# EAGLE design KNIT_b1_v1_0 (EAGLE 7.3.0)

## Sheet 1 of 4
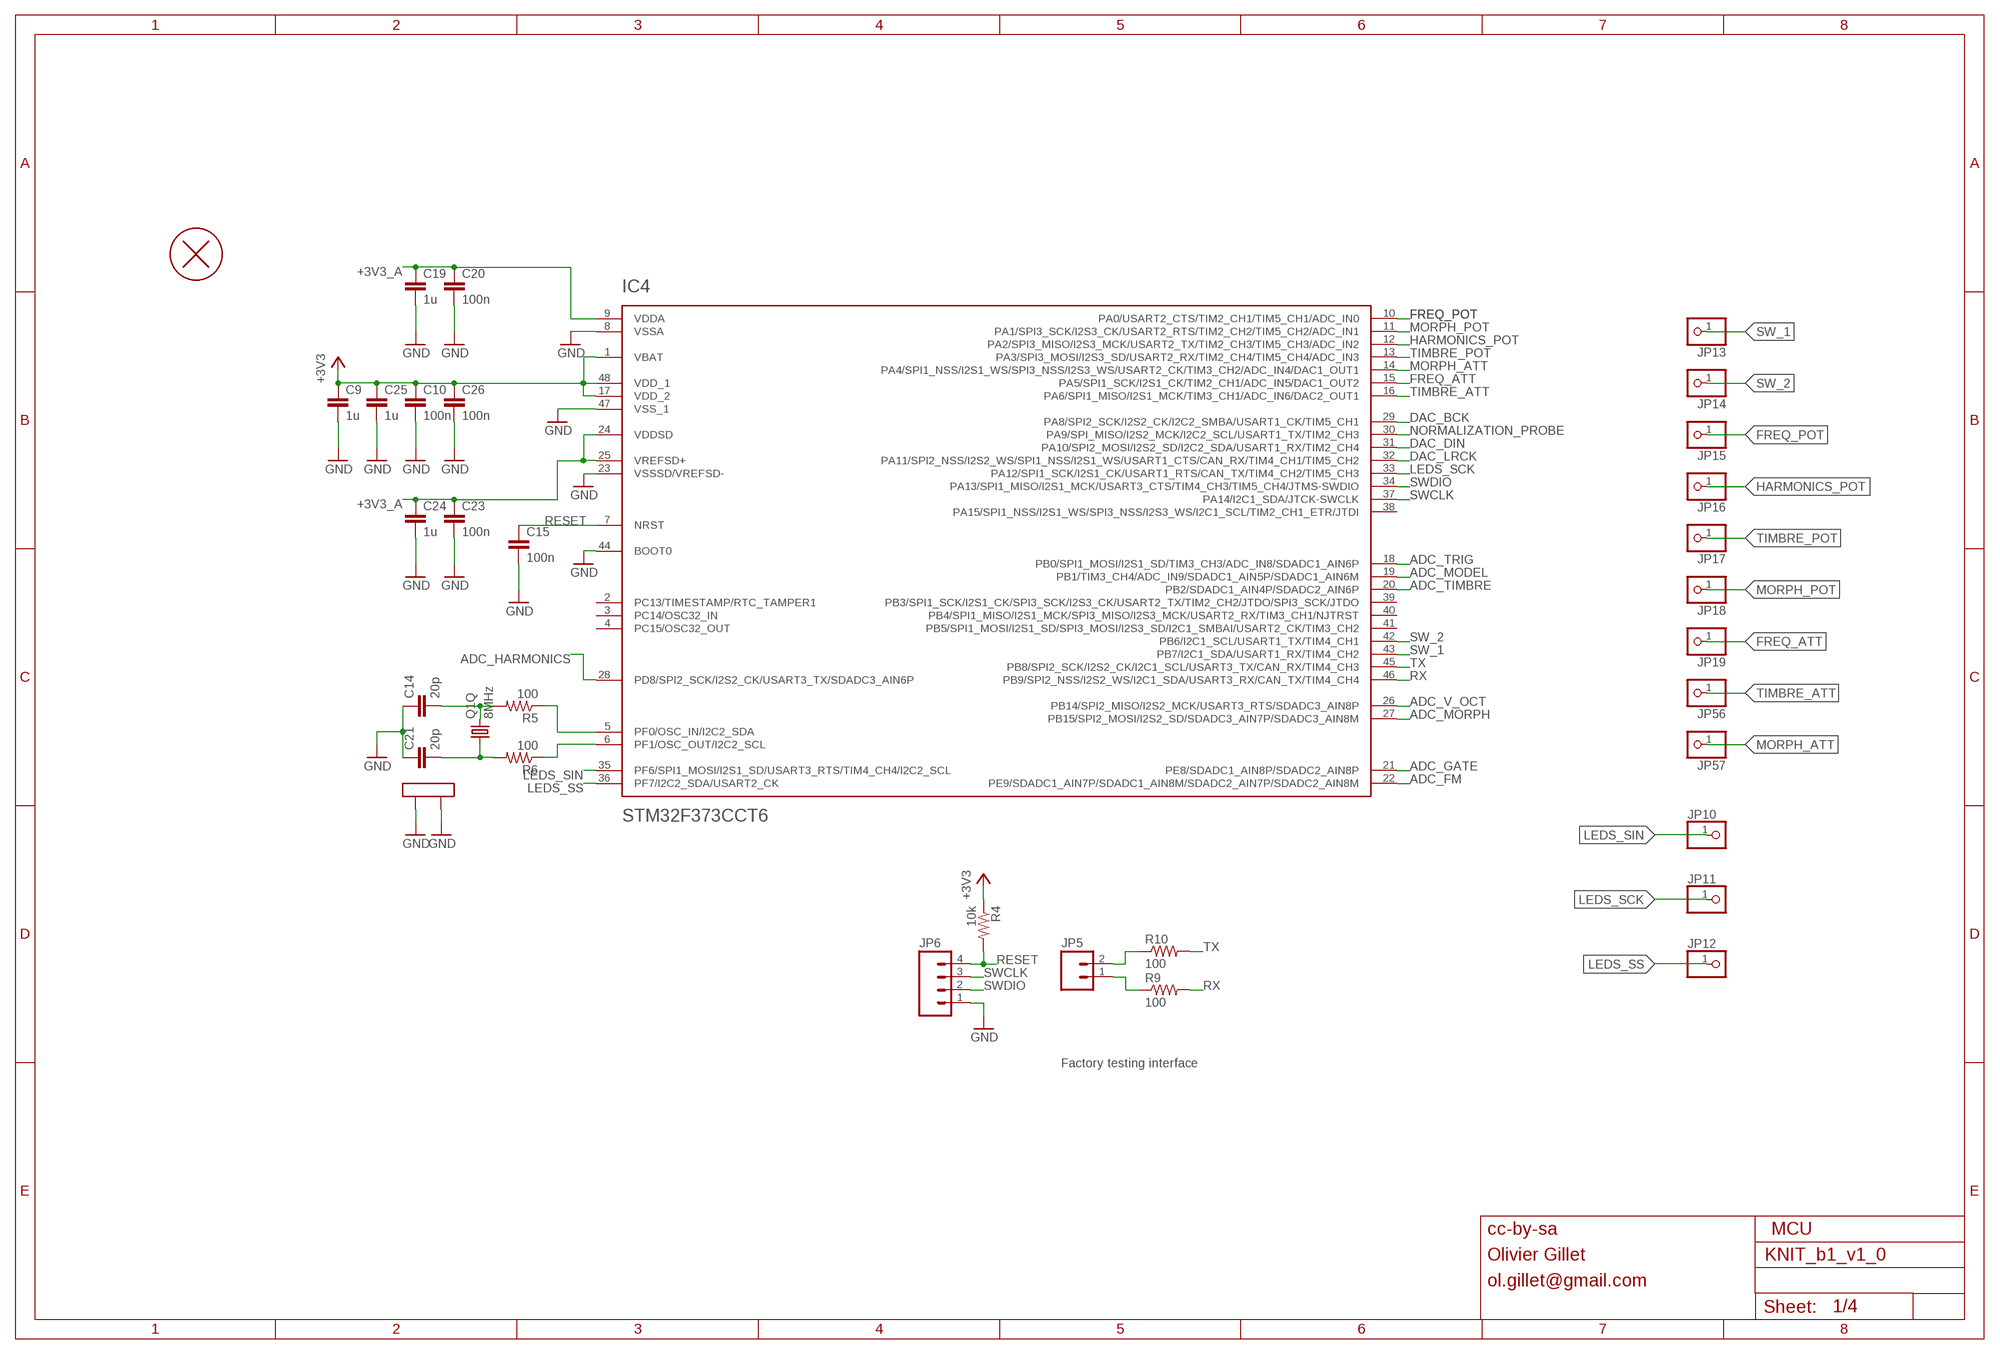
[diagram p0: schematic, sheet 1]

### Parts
C9  1u  CAPACITOR  [RESISTOR_0603]
C10  100n  CAPACITOR  [RESISTOR_0603]
C14  20p  CAPACITOR  [RESISTOR_0603]
C15  100n  CAPACITOR  [RESISTOR_0603]
C19  1u  CAPACITOR  [RESISTOR_0603]
C20  100n  CAPACITOR  [RESISTOR_0603]
C21  20p  CAPACITOR  [RESISTOR_0603]
C23  100n  CAPACITOR  [RESISTOR_0603]
C24  1u  CAPACITOR  [RESISTOR_0603]
C25  1u  CAPACITOR  [RESISTOR_0603]
C26  100n  CAPACITOR  [RESISTOR_0603]
H1  PCB_SCREW  [PCB_SCREW]
IC4  STM32F373CCT6  STM32F373C  [LQFP48]
JP5  M02PTH  [1X02]
JP6  M04PTH  [1X04]
JP10  PINHD-1X1  [1X01]
JP11  PINHD-1X1  [1X01]
JP12  PINHD-1X1  [1X01]
JP13  PINHD-1X1  [1X01]
JP14  PINHD-1X1  [1X01]
JP15  PINHD-1X1  [1X01]
JP16  PINHD-1X1  [1X01]
JP17  PINHD-1X1  [1X01]
JP18  PINHD-1X1  [1X01]
JP19  PINHD-1X1  [1X01]
JP56  PINHD-1X1  [1X01]
JP57  PINHD-1X1  [1X01]
Q1  8MHz  CRYSTAL  [CTS406]
R4  10k  RESISTOR  [RESISTOR_0603]
R5  100  RESISTOR  [RESISTOR_0603]
R6  100  RESISTOR  [RESISTOR_0603]
R9  100  RESISTOR  [RESISTOR_0603]
R10  100  RESISTOR  [RESISTOR_0603]

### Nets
+3V3: C9.1 C10.1 C25.1 C26.1 IC4.1(VBAT) IC4.17(VDD_2) IC4.48(VDD_1) R4.1 ; also sheet 3,4
+3V3_A: C19.1 C20.1 C23.1 C24.1 IC4.9(VDDA) IC4.24(VDDSD) IC4.25(VREFSD+) ; also sheet 2,3,4
ADC_FM: IC4.22(PE9/SDADC1_AIN7P/SDADC1_AIN8M/SDADC2_AIN7P/SDADC2_AIN8M) ; also sheet 2
ADC_GATE: IC4.21(PE8/SDADC1_AIN8P/SDADC2_AIN8P) ; also sheet 2
ADC_HARMONICS: IC4.28(PD8/SPI2_SCK/I2S2_CK/USART3_TX/SDADC3_AIN6P) ; also sheet 2
ADC_MODEL: IC4.19(PB1/TIM3_CH4/ADC_IN9/SDADC1_AIN5P/SDADC1_AIN6M) ; also sheet 2
ADC_MORPH: IC4.27(PB15/SPI2_MOSI/I2S2_SD/SDADC3_AIN7P/SDADC3_AIN8M) ; also sheet 2
ADC_TIMBRE: IC4.20(PB2/SDADC1_AIN4P/SDADC2_AIN6P) ; also sheet 2
ADC_TRIG: IC4.18(PB0/SPI1_MOSI/I2S1_SD/TIM3_CH3/ADC_IN8/SDADC1_AIN6P) ; also sheet 2
ADC_V_OCT: IC4.26(PB14/SPI2_MISO/I2S2_MCK/USART3_RTS/SDADC3_AIN8P) ; also sheet 2
DAC_BCK: IC4.29(PA8/SPI2_SCK/I2S2_CK/I2C2_SMBA/USART1_CK/TIM5_CH1) ; also sheet 3
DAC_DIN: IC4.31(PA10/SPI2_MOSI/I2S2_SD/I2C2_SDA/USART1_RX/TIM2_CH4) ; also sheet 3
DAC_LRCK: IC4.32(PA11/SPI2_NSS/I2S2_WS/SPI1_NSS/I2S1_WS/USART1_CTS/CAN_RX/TIM4_CH1/TIM5_CH2) ; also sheet 3
FREQ_ATT: IC4.15(PA5/SPI1_SCK/I2S1_CK/TIM2_CH1/ADC_IN5/DAC1_OUT2) JP19.1
FREQ_POT: IC4.10(PA0/USART2_CTS/TIM2_CH1/TIM5_CH1/ADC_IN0) JP15.1
GND: C9.2 C10.2 C14.1 C15.2 C19.2 C20.2 C21.1 C23.2 C24.2 C25.2 C26.2 IC4.8(VSSA) IC4.23(VSSSD/VREFSD-) IC4.44(BOOT0) IC4.47(VSS_1) JP6.1 Q1.2(LID1) Q1.4(LID2) ; also sheet 2,3,4
HARMONICS_POT: IC4.12(PA2/SPI3_MISO/I2S3_MCK/USART2_TX/TIM2_CH3/TIM5_CH3/ADC_IN2) JP16.1
LEDS_SCK: IC4.33(PA12/SPI1_SCK/I2S1_CK/USART1_RTS/CAN_TX/TIM4_CH2/TIM5_CH3) JP11.1
LEDS_SIN: IC4.35(PF6/SPI1_MOSI/I2S1_SD/USART3_RTS/TIM4_CH4/I2C2_SCL) JP10.1
LEDS_SS: IC4.36(PF7/I2C2_SDA/USART2_CK) JP12.1
MORPH_ATT: IC4.14(PA4/SPI1_NSS/I2S1_WS/SPI3_NSS/I2S3_WS/USART2_CK/TIM3_CH2/ADC_IN4/DAC1_OUT1) JP57.1
MORPH_POT: IC4.11(PA1/SPI3_SCK/I2S3_CK/USART2_RTS/TIM2_CH2/TIM5_CH2/ADC_IN1) JP18.1
N$7: IC4.5(PF0/OSC_IN/I2C2_SDA) R5.1
N$8: IC4.6(PF1/OSC_OUT/I2C2_SCL) R6.1
N$29: C14.2 Q1.3 R5.2
N$33: JP5.2 R10.1
N$35: C21.2 Q1.1 R6.2
N$51: JP5.1 R9.1
NORMALIZATION_PROBE: IC4.30(PA9/SPI_MISO/I2S2_MCK/I2C2_SCL/USART1_TX/TIM2_CH3) ; also sheet 2
RESET: C15.1 IC4.7(NRST) JP6.4 R4.2
RX: IC4.46(PB9/SPI2_NSS/I2S2_WS/I2C1_SDA/USART3_RX/CAN_TX/TIM4_CH4) R9.2
SW_1: IC4.43(PB7/I2C1_SDA/USART1_RX/TIM4_CH2) JP13.1
SW_2: IC4.42(PB6/I2C1_SCL/USART1_TX/TIM4_CH1) JP14.1
SWCLK: IC4.37(PA14/I2C1_SDA/JTCK-SWCLK) JP6.3
SWDIO: IC4.34(PA13/SPI1_MISO/I2S1_MCK/USART3_CTS/TIM4_CH3/TIM5_CH4/JTMS-SWDIO) JP6.2
TIMBRE_ATT: IC4.16(PA6/SPI1_MISO/I2S1_MCK/TIM3_CH1/ADC_IN6/DAC2_OUT1) JP56.1
TIMBRE_POT: IC4.13(PA3/SPI3_MOSI/I2S3_SD/USART2_RX/TIM2_CH4/TIM5_CH4/ADC_IN3) JP17.1
TX: IC4.45(PB8/SPI2_SCK/I2S2_CK/I2C1_SCL/USART3_TX/CAN_RX/TIM4_CH3) R10.2
Unconnected: IC4.2(PC13/TIMESTAMP/RTC_TAMPER1) IC4.3(PC14/OSC32_IN) IC4.4(PC15/OSC32_OUT) IC4.38(PA15/SPI1_NSS/I2S1_WS/SPI3_NSS/I2S3_WS/I2C1_SCL/TIM2_CH1_ETR/JTDI) IC4.39(PB3/SPI1_SCK/I2S1_CK/SPI3_SCK/I2S3_CK/USART2_TX/TIM2_CH2/JTDO/SPI3_SCK/JTDO) IC4.40(PB4/SPI1_MISO/I2S1_MCK/SPI3_MISO/I2S3_MCK/USART2_RX/TIM3_CH1/NJTRST) IC4.41(PB5/SPI1_MOSI/I2S1_SD/SPI3_MOSI/I2S3_SD/I2C1_SMBAI/USART2_CK/TIM3_CH2)

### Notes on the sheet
- Factory testing interface
- cc-by-sa | MCU
- Olivier Gillet
- ol.gillet@gmail.com

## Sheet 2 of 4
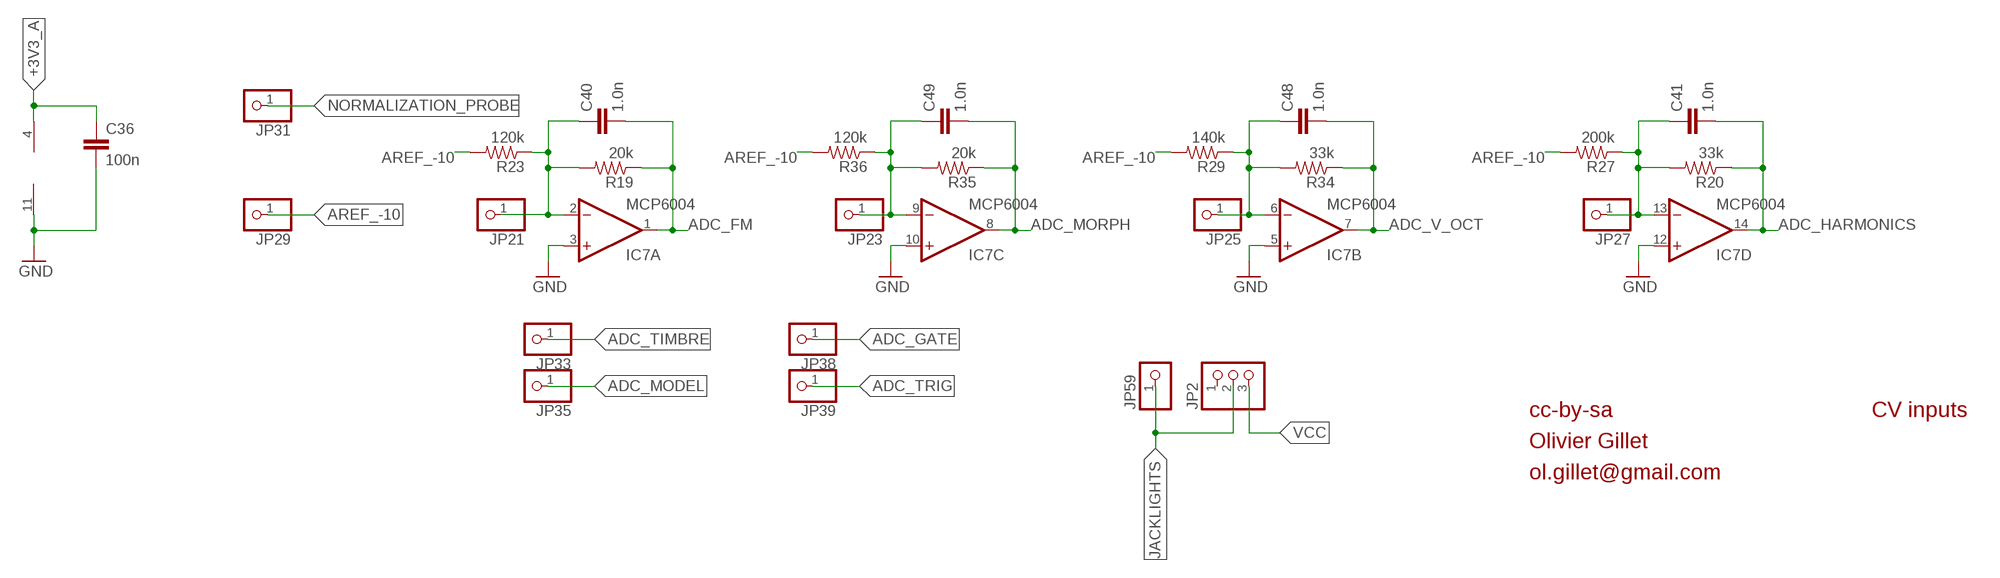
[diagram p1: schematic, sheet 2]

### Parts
C36  100n  CAPACITOR  [RESISTOR_0603]
C40  1.0n  CAPACITOR  [RESISTOR_0603]
C41  1.0n  CAPACITOR  [RESISTOR_0603]
C48  1.0n  CAPACITOR  [RESISTOR_0603]
C49  1.0n  CAPACITOR  [RESISTOR_0603]
IC7  MCP6004  TL074PW  [TSSOP14_065]
JP2  PINHD-1X3  [1X03]
JP21  PINHD-1X1  [1X01]
JP23  PINHD-1X1  [1X01]
JP25  PINHD-1X1  [1X01]
JP27  PINHD-1X1  [1X01]
JP29  PINHD-1X1  [1X01]
JP31  PINHD-1X1  [1X01]
JP33  PINHD-1X1  [1X01]
JP35  PINHD-1X1  [1X01]
JP38  PINHD-1X1  [1X01]
JP39  PINHD-1X1  [1X01]
JP59  PINHD-1X1  [1X01]
R19  20k  RESISTOR  [RESISTOR_0603]
R20  33k  RESISTOR  [RESISTOR_0603]
R23  120k  RESISTOR  [RESISTOR_0603]
R27  200k  RESISTOR  [RESISTOR_0603]
R29  140k  RESISTOR  [RESISTOR_0603]
R34  33k  RESISTOR  [RESISTOR_0603]
R35  20k  RESISTOR  [RESISTOR_0603]
R36  120k  RESISTOR  [RESISTOR_0603]

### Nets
+3V3_A: C36.1 IC7.4(P:V+) ; also sheet 1,3,4
ADC_FM: C40.2 IC7.1(A:OUT) R19.1 ; also sheet 1
ADC_GATE: JP38.1 ; also sheet 1
ADC_HARMONICS: C41.2 IC7.14(D:OUT) R20.1 ; also sheet 1
ADC_MODEL: JP35.1 ; also sheet 1
ADC_MORPH: C49.2 IC7.8(C:OUT) R35.1 ; also sheet 1
ADC_TIMBRE: JP33.1 ; also sheet 1
ADC_TRIG: JP39.1 ; also sheet 1
ADC_V_OCT: C48.2 IC7.7(B:OUT) R34.1 ; also sheet 1
AREF_-10: JP29.1 R23.2 R27.2 R29.2 R36.2 ; also sheet 4
GND: C36.2 IC7.3(A:+IN) IC7.5(B:+IN) IC7.10(C:+IN) IC7.11(P:V-) IC7.12(D:+IN) ; also sheet 1,3,4
JACKLIGHTS: JP2.2 JP59.1
N$30: C48.1 IC7.6(B:-IN) JP25.1 R29.1 R34.2
N$32: C49.1 IC7.9(C:-IN) JP23.1 R35.2 R36.1
N$34: C40.1 IC7.2(A:-IN) JP21.1 R19.2 R23.1
N$41: C41.1 IC7.13(D:-IN) JP27.1 R20.2 R27.1
NORMALIZATION_PROBE: JP31.1 ; also sheet 1
VCC: JP2.3 ; also sheet 3,4
Unconnected: JP2.1

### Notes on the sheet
- cc-by-sa | CV inputs
- Olivier Gillet
- ol.gillet@gmail.com

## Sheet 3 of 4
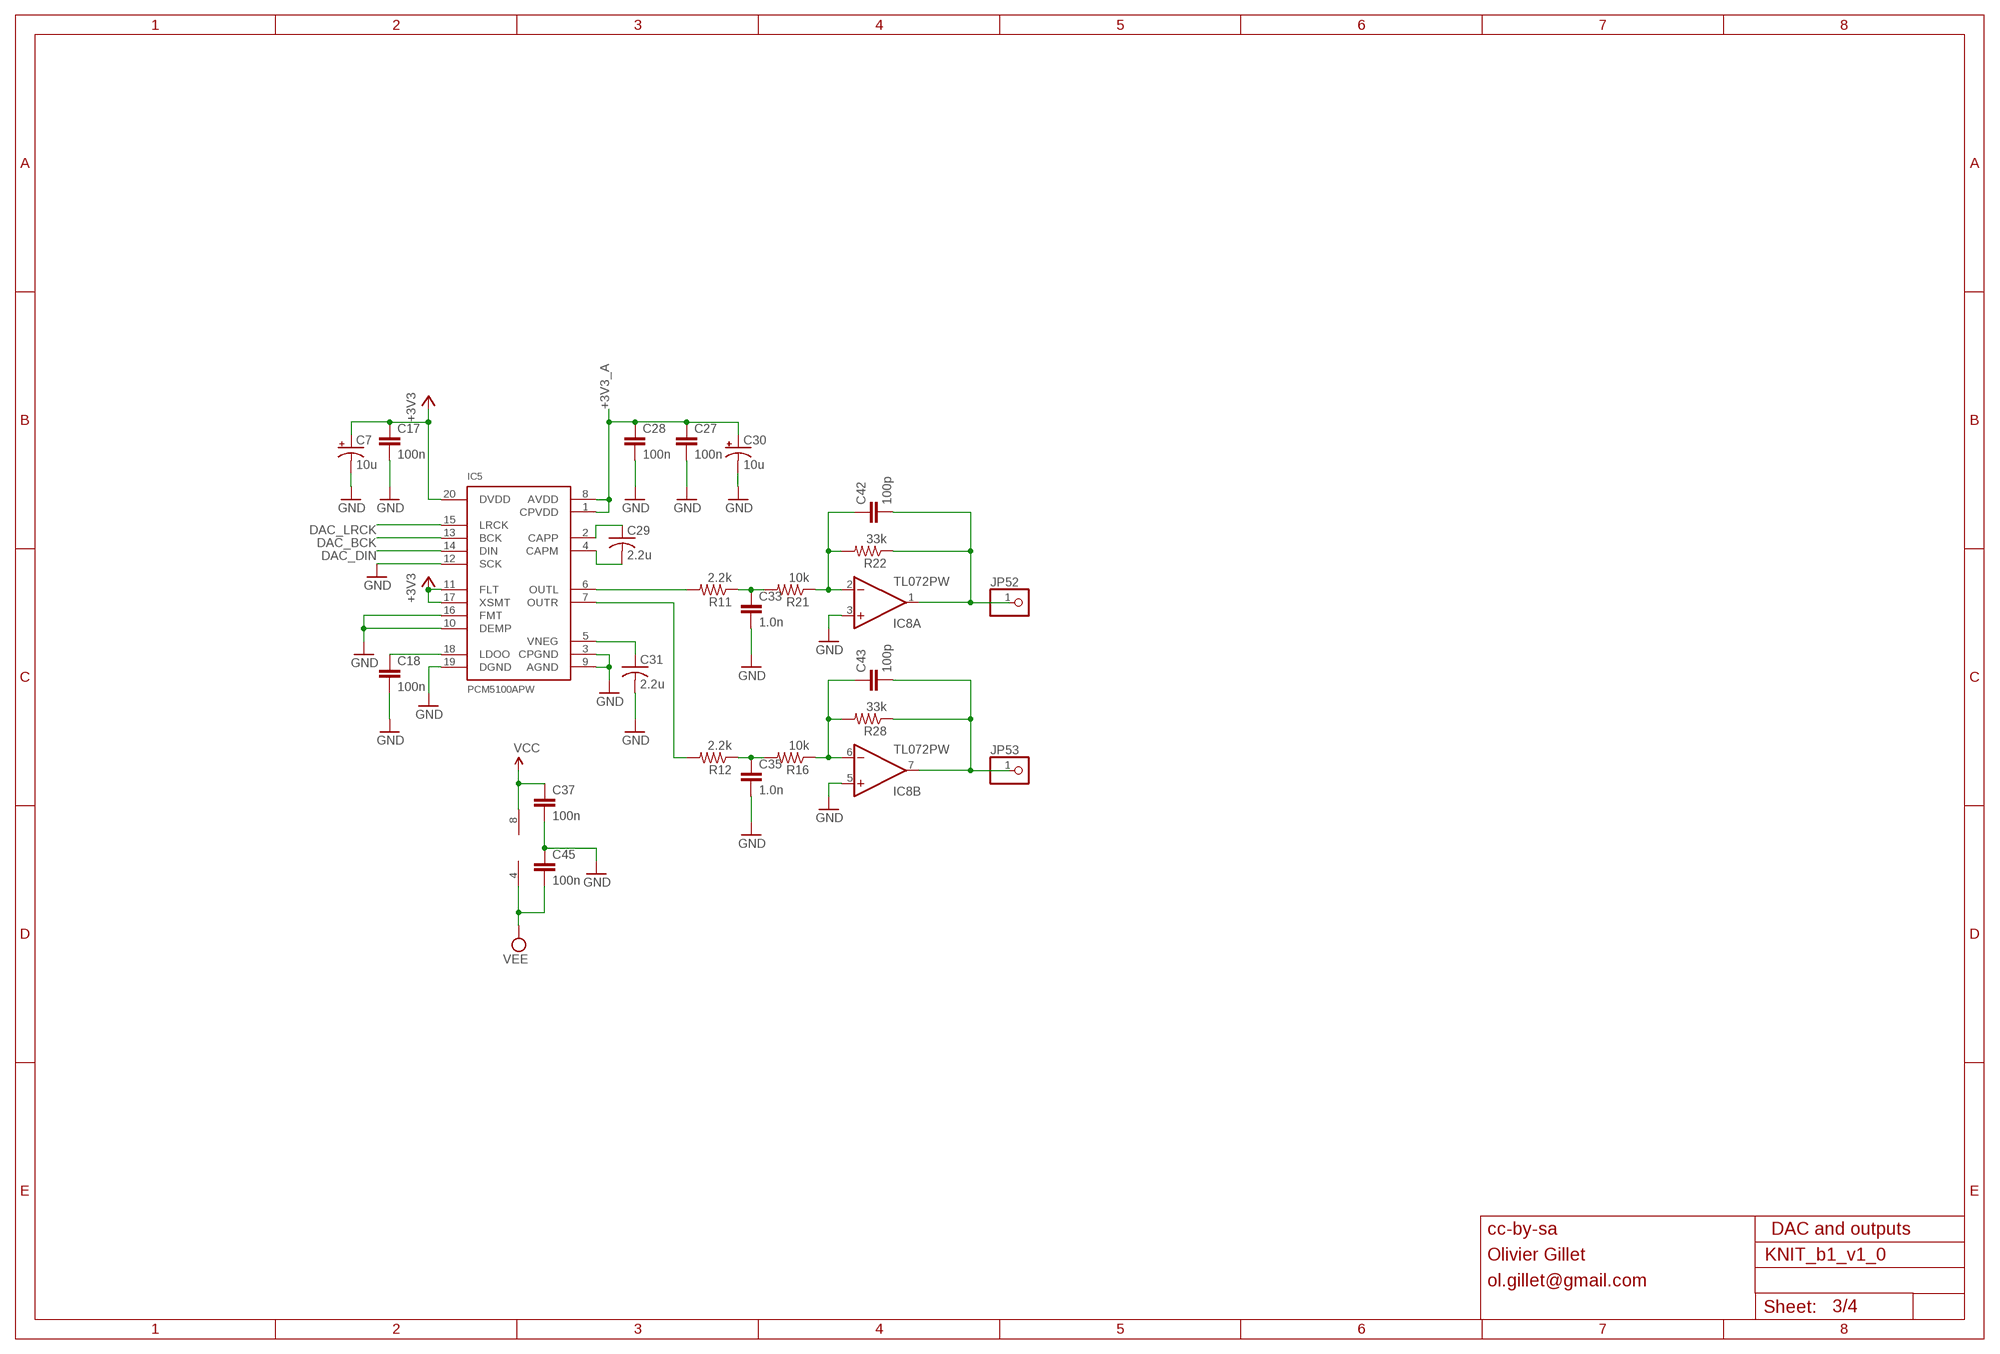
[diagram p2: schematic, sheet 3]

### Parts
C7  10u  CAP_POL  [PANASONIC_B]
C17  100n  CAPACITOR  [RESISTOR_0603]
C18  100n  CAPACITOR  [RESISTOR_0603]
C27  100n  CAPACITOR  [RESISTOR_0603]
C28  100n  CAPACITOR  [RESISTOR_0603]
C29  2.2u  C-USC0805  [C0805]
C30  10u  CAP_POL  [PANASONIC_B]
C31  2.2u  C-USC0805  [C0805]
C33  1.0n  CAPACITOR  [RESISTOR_0603]
C35  1.0n  CAPACITOR  [RESISTOR_0603]
C37  100n  CAPACITOR  [RESISTOR_0603]
C42  100p  CAPACITOR  [RESISTOR_0603]
C43  100p  CAPACITOR  [RESISTOR_0603]
C45  100n  CAPACITOR  [RESISTOR_0603]
IC5  PCM5100APW  PCM5100PW  [SSOP20]
IC8  TL072PW  [TSSOP08]
JP52  PINHD-1X1  [1X01]
JP53  PINHD-1X1  [1X01]
R11  2.2k  RESISTOR  [RESISTOR_0603]
R12  2.2k  RESISTOR  [RESISTOR_0603]
R16  10k  RESISTOR  [RESISTOR_0603]
R21  10k  RESISTOR  [RESISTOR_0603]
R22  33k  RESISTOR  [RESISTOR_0603]
R28  33k  RESISTOR  [RESISTOR_0603]

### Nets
+3V3: C7.+ C17.1 IC5.11(FLT) IC5.17(XSMT) IC5.20(DVDD) ; also sheet 1,4
+3V3_A: C27.1 C28.1 C30.+ IC5.1(CPVDD) IC5.8(AVDD) ; also sheet 1,2,4
DAC_BCK: IC5.13(BCK) ; also sheet 1
DAC_DIN: IC5.14(DIN) ; also sheet 1
DAC_LRCK: IC5.15(LRCK) ; also sheet 1
GND: C7.- C17.2 C18.2 C27.2 C28.2 C30.- C31.2 C33.2 C35.2 C37.2 C45.1 IC5.3(CPGND) IC5.9(AGND) IC5.10(DEMP) IC5.12(SCK) IC5.16(FMT) IC5.19(DGND) IC8.3(A:+IN) IC8.5(B:+IN) ; also sheet 1,2,4
N$6: C29.1 IC5.2(CAPP)
N$16: C29.2 IC5.4(CAPM)
N$43: IC5.6(OUTL) R11.2
N$46: C33.1 R11.1 R21.2
N$47: C35.1 R12.1 R16.2
N$48: C31.1 IC5.5(VNEG)
N$54: C18.1 IC5.18(LDOO)
N$55: IC5.7(OUTR) R12.2
N$58: C43.1 IC8.6(B:-IN) R16.1 R28.2
N$60: C43.2 IC8.7(B:OUT) JP53.1 R28.1
N$62: C42.1 IC8.2(A:-IN) R21.1 R22.2
N$63: C42.2 IC8.1(A:OUT) JP52.1 R22.1
VCC: C37.1 IC8.8(P:V+) ; also sheet 2,4
VEE: C45.2 IC8.4(P:V-) ; also sheet 4

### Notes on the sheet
- cc-by-sa | DAC and outputs
- Olivier Gillet
- ol.gillet@gmail.com

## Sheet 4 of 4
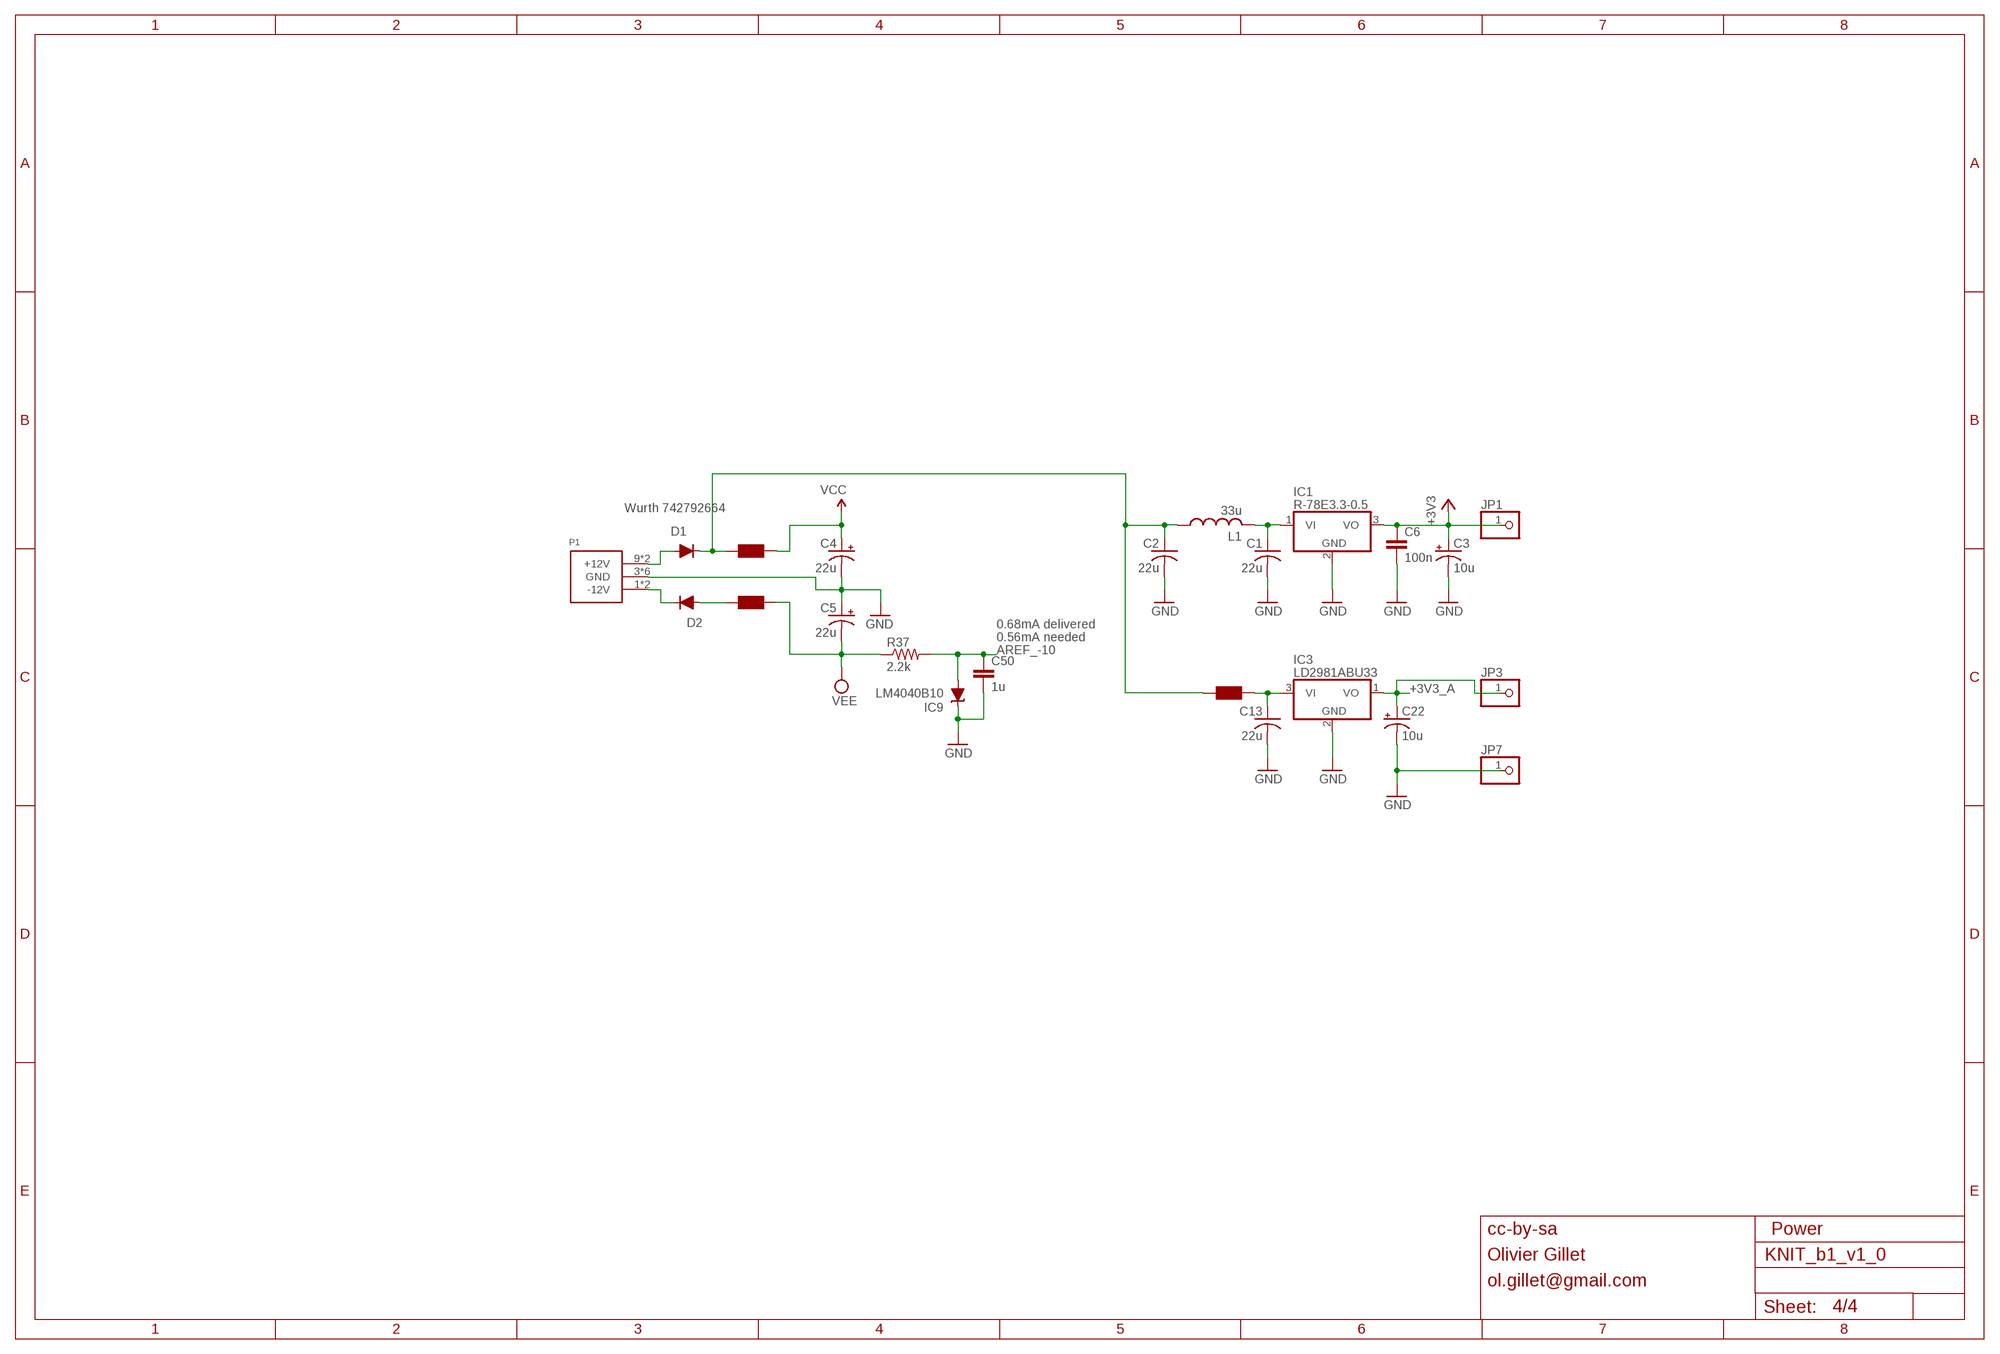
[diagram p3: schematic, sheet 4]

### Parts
C1  22u  C-USC1206  [C1206]
C2  22u  C-USC1206  [C1206]
C3  10u  CAP_POL  [PANASONIC_B]
C4  22u  CAP_POL  [PANASONIC_B]
C5  22u  CAP_POL  [PANASONIC_B]
C6  100n  CAPACITOR  [RESISTOR_0603]
C13  22u  C-USC1206  [C1206]
C22  10u  CAP_POL  [PANASONIC_B]
C50  1u  CAPACITOR  [RESISTOR_0603]
D1  1N5819HW  DIODE  [SOD123]
D2  1N5819HW  DIODE  [SOD123]
F1  FERRITE-BEAD  [RESISTOR_0603]
F2  FERRITE-BEAD  [RESISTOR_0603]
F3  FERRITE-BEAD  [RESISTOR_0603]
IC1  R-78E3.3-0.5  WE173950378  [WE78]
IC3  LD2981ABU33  LD2981ABU  [SOT89]
IC9  LM4040B10  LM4041B12DBZ  [DBZ_R-PDSO-G3]
JP1  PINHD-1X1  [1X01]
JP3  PINHD-1X1  [1X01]
JP7  PINHD-1X1  [1X01]
L1  33u  L-USL2012C  [L2012C]
P1  POWER_SIMPLE10  [POWER_10]
R37  2.2k  RESISTOR  [RESISTOR_0603]

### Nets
+3V3: C3.+ C6.1 IC1.3(VO) JP1.1 ; also sheet 1,3
+3V3_A: C22.+ IC3.1(VO) JP3.1 ; also sheet 1,2,3
AREF_-10: C50.1 IC9.2(A) R37.2 ; also sheet 2
GND: C1.2 C2.2 C3.- C4.- C5.+ C6.2 C13.2 C22.- C50.2 IC1.2(GND) IC3.2(GND) IC9.1(C) JP7.1 P1.3(GND) P1.4(GND) P1.5(GND) P1.6(GND) P1.7(GND) P1.8(GND) ; also sheet 1,2,3
N$1: C1.1 IC1.1(VI) L1.2
N$2: D1.+ P1.9(+12V) P1.10(+12V)
N$3: D2.- P1.1(-12V) P1.2(-12V)
N$38: D2.+ F2.2
N$40: C2.1 D1.- F1.2 F3.2 L1.1
N$42: C13.1 F3.1 IC3.3(VI)
VCC: C4.+ F1.1 ; also sheet 2,3
VEE: C5.- F2.1 R37.1 ; also sheet 3

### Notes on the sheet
- Wurth 742792664
- 0.68mA delivered
- 0.56mA needed
- cc-by-sa | Power
- Olivier Gillet
- ol.gillet@gmail.com

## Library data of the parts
C1 C2 C13 C29 C31 = rcl:C-US: CAPACITOR, American symbol
C3-C5 C7 C22 C30 = parts_aman:CAP_POL
C6 C9 C10 C14 C15 C17-C21 C23-C28 C33 C35-C37 C40-C43 C45 C48-C50 = parts_aman:CAPACITOR
D1 D2 = parts_aman:DIODE
F1-F3 = parts_aman:FERRITE-BEAD
H1 = parts_aman:PCB_SCREW
IC1 = og-vreg:WE173950378
IC3 = og-vreg:LD2981
IC4 = og-stm32f2:STM32F373C
IC5 = og-dac:PCM5100
IC7 = og-linear:TL074: OP AMP
IC8 = og-linear:TL072: OP AMP
IC9 = texas:LM4041: PRECISION MICROPOWER SHUNT VOLTAGE REFERENCE
JP1 JP3 JP7 JP10-JP19 JP21 JP23 JP25 JP27 JP29 JP31 JP33 JP35 JP38 JP39 JP52 JP53 JP56 JP57 JP59 = parts_aman:PINHD-1X1: PIN HEADER
JP2 = parts_aman:PINHD-1X3: PIN HEADER
JP5 = SparkFun:M02: Header 2
JP6 = SparkFun:M04: Header 4 Standard 4-pin 0.1" header. Use with straight break away headers (SKU : PRT-00116), right angle break away headers (PRT-00553), swiss pins (PRT-00743), machine pins (PRT-00117), and female headers (PRT-00115). Molex polarized connector foot print use with SKU : PRT-08231 with associated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
L1 = og-rcl:L-US
P1 = parts_aman:POWER_SIMPLE
Q1 = og-crystal:CRYSTAL: Crystal with 2 extra terminals for the metal LID (Abracon ABMM2 for example)
R4-R6 R9-R12 R16 R19-R23 R27-R29 R34-R37 = parts_aman:RESISTOR

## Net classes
0 default: width 0.152 mm, drill 0.305 mm, clearance 0.152 mm

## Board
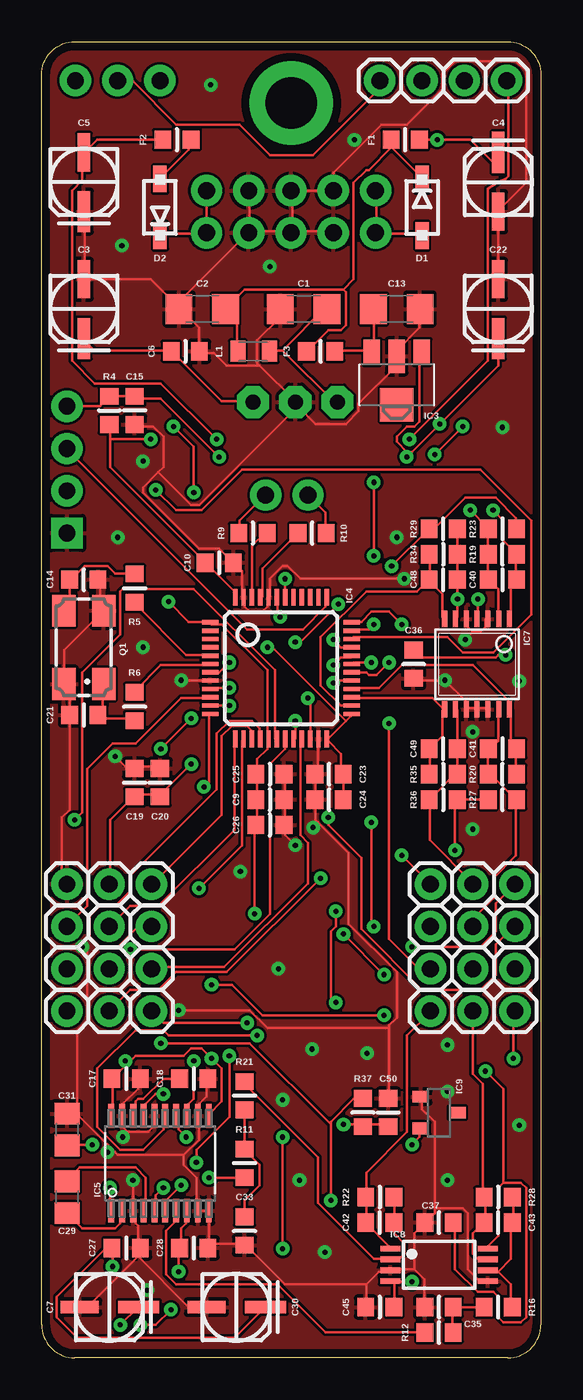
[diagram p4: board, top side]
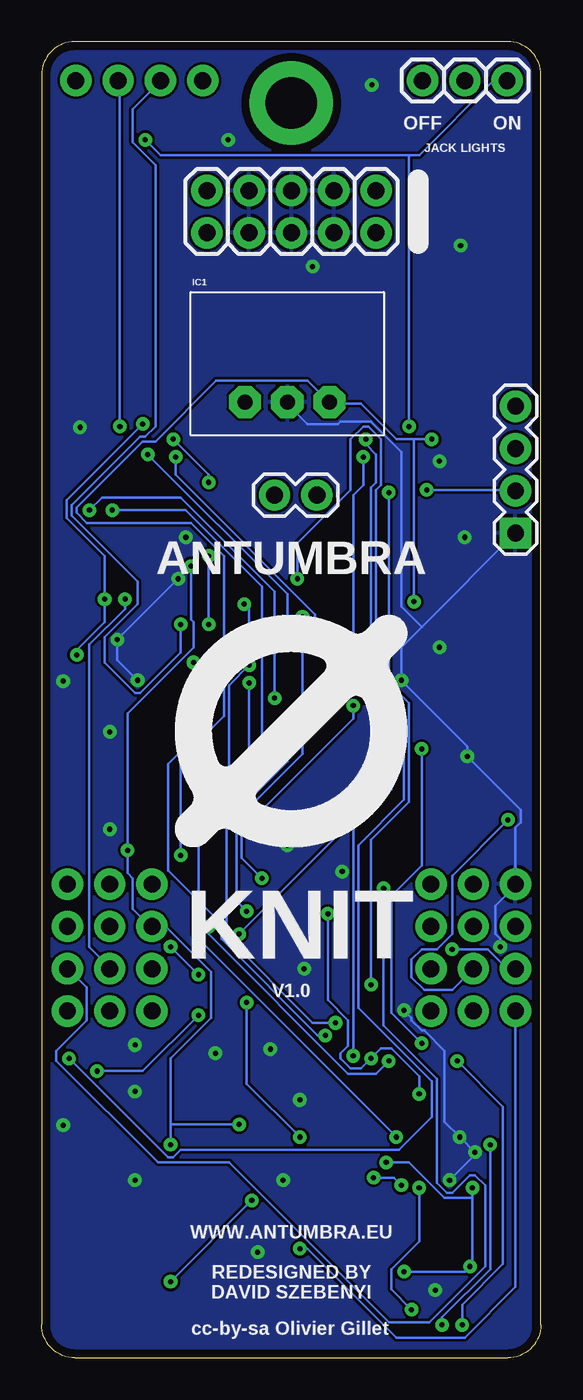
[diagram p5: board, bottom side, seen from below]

Size 30 x 79.04 mm. Coordinates in mm from the lower left corner, seen from the top.
Outline: 28,0 2,0 arc-90 0,2 0,77.04 arc-90 2,79.04 28,79.04 arc-90 30,77.04 30,2 arc-90 28,0
Copper layers (1*16): Top 0.035mm / dielectric 1.5mm / Bottom 0.035mm
Design rules "PCBCart-Standard *": minimum track width 6mil, minimum drill 12mil, track to track 6mil, track to pad 6mil, pad to pad 6mil, via to via 6mil, smd to smd 6mil, copper to edge 20mil, drill to drill 8mil, minimum pad ring 8mil, minimum via ring 10mil, stop-mask expansion 3mil, vias tented up to drill 25mil, thermal gap 8mil

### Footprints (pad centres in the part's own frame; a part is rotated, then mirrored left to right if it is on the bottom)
C1206 = smd 1.6 x 1.8: 1 -1.4,0; 2 1.4,0
PANASONIC_B = smd 2.464 x 0.762: + 1.778,0 | smd 2.286 x 0.762: - -1.778,0
RESISTOR_0603 = smd 1 x 1.1: 1 -0.85,0; 2 0.85,0
C0805 = smd 1.3 x 1.5: 1 -0.95,0; 2 0.95,0
SOD123 = smd 1.6 x 0.8: + 1.7,0; - -1.7,0
PCB_SCREW = drill 3.1 pad 5: P$1 0,0
WE78 = drill 0.9 pad 1.93 octagon: 1 -2.54,0; 2 0,0; 3 2.54,0
SOT89 = smd 1 x 1.5: 1 -1.499,-1.981; 3 1.499,-1.981 | smd 1 x 2: 2 0,-1.727 | smd 2 x 2: 2@1 0,1.194
LQFP48 = smd 0.254 x 1: 1 -2.75,-4.25; 2 -2.25,-4.25; 3 -1.75,-4.25; 4 -1.25,-4.25; 5 -0.75,-4.25; 6 -0.25,-4.25; 7 0.25,-4.25; 8 0.75,-4.25; 9 1.25,-4.25; 10 1.75,-4.25; 11 2.25,-4.25; 12 2.75,-4.25; 25 2.75,4.25; 26 2.25,4.25; 27 1.75,4.25; 28 1.25,4.25; 29 0.75,4.25; 30 0.25,4.25; 31 -0.25,4.25; 32 -0.75,4.25; 33 -1.25,4.25; 34 -1.75,4.25; 35 -2.25,4.25; 36 -2.75,4.25 | smd 1 x 0.254: 13 4.25,-2.75; 14 4.25,-2.25; 15 4.25,-1.75; 16 4.25,-1.25; 17 4.25,-0.75; 18 4.25,-0.25; 19 4.25,0.25; 20 4.25,0.75; 21 4.25,1.25; 22 4.25,1.75; 23 4.25,2.25; 24 4.25,2.75; 37 -4.25,2.75; 38 -4.25,2.25; 39 -4.25,1.75; 40 -4.25,1.25; 41 -4.25,0.75; 42 -4.25,0.25; 43 -4.25,-0.25; 44 -4.25,-0.75; 45 -4.25,-1.25; 46 -4.25,-1.75; 47 -4.25,-2.25; 48 -4.25,-2.75
SSOP20 = smd 1.422 x 0.356: 1 -2.845,2.936; 2 -2.845,2.276; 3 -2.845,1.615; 4 -2.845,0.98; 5 -2.845,0.32; 6 -2.845,-0.315; 7 -2.845,-0.98; 8 -2.845,-1.615; 9 -2.845,-2.276; 10 -2.845,-2.936; 11 2.845,-2.936; 12 2.845,-2.276; 13 2.845,-1.615; 14 2.845,-0.98; 15 2.845,-0.315; 16 2.845,0.32; 17 2.845,0.98; 18 2.845,1.615; 19 2.845,2.276; 20 2.845,2.936
TSSOP14_065 = smd 0.305 x 0.991: 1 -1.95,-2.718; 2 -1.3,-2.718; 3 -0.65,-2.718; 4 0,-2.718; 5 0.65,-2.718; 6 1.3,-2.718; 7 1.95,-2.718; 8 1.95,2.718; 9 1.3,2.718; 10 0.65,2.718; 11 0,2.718; 12 -0.65,2.718; 13 -1.3,2.718; 14 -1.95,2.718
TSSOP08 = smd 0.35 x 1.2: 1 -0.975,-2.925; 2 -0.325,-2.925; 3 0.325,-2.925; 4 0.975,-2.925; 5 0.975,2.925; 6 0.325,2.925; 7 -0.325,2.925; 8 -0.975,2.925
DBZ_R-PDSO-G3 = smd 0.7 x 1: 1 -0.95,-1.1; 2 0.95,-1.1; 3 0,1.1
1X01 = drill 1.016 pad 1.88: 1 0,0
1X03 = drill 1.016 pad 1.88: 1 -2.54,0; 2 0,0; 3 2.54,0
1X02 = drill 1.016 pad 1.88: 1 0,0; 2 2.54,0
1X04 = drill 1.016 pad 1.88 square: 1 0,0 | drill 1.016 pad 1.88: 2 2.54,0; 3 5.08,0; 4 7.62,0
L2012C = smd 0.9 x 1.25: 1 -0.9,0; 2 1,0
POWER_10 = drill 1.016 pad 1.88: 1 -5.08,-1.27; 2 -5.08,1.27; 3 -2.54,-1.27; 4 -2.54,1.27; 5 0,-1.27; 6 0,1.27; 7 2.54,-1.27; 8 2.54,1.27; 9 5.08,-1.27; 10 5.08,1.27
CTS406 = smd 1.9 x 1.4: 1 -2.2,-1.2; 2 2.2,-1.2; 3 2.2,1.2; 4 -2.2,1.2

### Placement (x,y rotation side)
C1  15.75,62.99 180 top
C2  9.65,62.99 180 top
C3  2.54,62.99 270 top
C4  27.43,70.61 90 top
C5  2.54,70.61 270 top
C6  8.64,60.45 0 top
C7  4.06,3.05 0 top
C9  13.72,33.53 0 top
C10  10.67,47.75 0 top
C13  21.34,62.99 0 top
C14  2.54,46.74 180 top
C15  5.59,56.9 270 top
C17  5.08,16.76 0 top
C18  9.14,16.76 0 top
C19  5.59,34.54 90 top
C20  7.11,34.54 90 top
C21  2.54,38.61 0 top
C22  27.43,62.99 270 top
C23  17.27,35.05 180 top
C24  17.27,33.53 180 top
C25  13.72,35.05 0 top
C26  13.72,32 0 top
C27  5.08,6.6 0 top
C28  9.14,6.6 0 top
C29  1.52,9.65 90 top
C30  11.68,3.05 0 top
C31  1.52,13.72 90 top
C33  12.19,7.62 270 top
C35  23.88,3.05 180 top
C36  22.35,41.66 270 top
C37  23.88,8.13 180 top
C40  27.69,46.74 0 top
C41  27.69,36.58 0 top
C42  20.32,8.13 180 top
C43  27.43,8.13 180 top
C45  20.32,3.05 0 top
C48  24.13,46.74 180 top
C49  24.13,36.58 180 top
C50  20.83,14.73 90 top
D1  22.86,69.09 270 top
D2  7.11,69.09 90 top
F1  21.84,73.15 180 top
F2  8.13,73.15 0 top
F3  16.76,60.45 180 top
H1  15,75.36 0 top
IC1  15.24,57.4 0 bottom
IC3  21.34,58.42 180 top
IC4  14.38,41.42 270 top
IC5  7.11,11.68 90 top
IC7  26.16,41.66 180 top
IC8  23.88,5.59 270 top
IC9  23.88,14.73 270 top
JP1  23.37,28.45 0 top
JP2  4.57,76.71 0 bottom
JP3  4.06,28.45 0 top
JP5  13.46,51.82 180 bottom
JP6  1.52,49.53 90 bottom
JP7  1.52,28.45 0 top
JP10  27.94,76.71 0 top
JP11  25.4,76.71 0 top
JP12  22.86,76.71 0 top
JP13  4.06,20.83 0 top
JP14  28.45,20.83 0 top
JP15  1.52,25.91 0 top
JP16  28.45,28.45 0 top
JP17  4.06,25.91 0 top
JP18  28.45,25.91 0 top
JP19  6.6,28.45 0 top
JP21  6.6,20.83 0 top
JP23  25.91,28.45 0 top
JP25  25.91,23.37 0 top
JP27  25.91,25.91 0 top
JP29  23.37,25.91 0 top
JP31  23.37,23.37 0 top
JP33  1.52,20.83 0 top
JP35  1.52,23.37 0 top
JP38  6.6,23.37 0 top
JP39  4.06,23.37 0 top
JP52  23.37,20.83 0 top
JP53  25.91,20.83 0 top
JP56  6.6,25.91 0 top
JP57  28.45,23.37 0 top
JP59  20.32,76.71 0 top
L1  12.7,60.45 0 top
P1  14.99,68.83 180 bottom
Q1  2.54,42.67 90 top
R4  4.06,56.9 90 top
R5  5.59,46.23 90 top
R6  5.59,39.12 270 top
R9  12.7,49.53 0 top
R10  16.26,49.53 180 top
R11  12.19,11.68 270 top
R12  23.88,1.52 180 top
R16  27.43,3.05 180 top
R19  27.69,48.26 180 top
R20  27.69,35.05 180 top
R21  12.19,15.75 270 top
R22  20.32,9.65 0 top
R23  27.69,49.78 0 top
R27  27.69,33.53 180 top
R28  27.43,9.65 0 top
R29  24.13,49.78 180 top
R34  24.13,48.26 0 top
R35  24.13,35.05 0 top
R36  24.13,33.53 0 top
R37  19.3,14.73 270 top
U$1  [LOGO_14]  15,37.65 0 bottom

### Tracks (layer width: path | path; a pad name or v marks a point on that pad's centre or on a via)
+3V3  (via drill 0.3)
  Top 0.152: 12.95,33.53 12.95,32 C26.1 12.8,32 v12.8,26.67 | 12.95,33.53 12.95,35.05 | 12.95,33.53 C9.1 | 12.95,35.05 12.95,35.97 13.56,36.58 13.56,37.03 IC4.17 13.56,37.19 13.56,41.3 10.82,44.04 10.21,44.04 IC4.1 10.06,44.2 8.84,44.2 v7.62,45.41 | 12.95,35.05 C25.1 | 4.27,16.76 4.27,14.63 IC5.20 | v7.32,15.85 6.86,15.85 6.25,15.24 6.25,14.63 IC5.17 | IC5.11 10.06,14.63 10.82,15.39 10.82,17.37 v10.21,17.98 9.6,18.59 8.99,18.59 8.53,18.14 5.64,18.14 5.18,17.68 | 5.18,17.68 4.27,16.76 | 4.27,16.76 C17.1 | v4.72,1.98 5.79,3.05 C7.+ | 5.18,17.68 v5.03,17.83 | IC4.48 11.58,45.72 11.58,46.02 9.91,47.7 C10.1 9.75,47.85 4.12,53.49 4.12,55.17 | 4.12,55.17 4.12,55.93 R4.1 | C3.+ 2.59,61.11 3.2,60.5 7.77,60.5 C6.1 7.92,60.35 10.82,57.45 12.65,57.45 IC1.3 | v21.64,30.18 JP1.1 | v6.55,55.17 4.12,55.17
  Bottom 0.152: v7.32,15.85 7.32,16.92 8.99,18.59 9.6,18.59 v10.21,17.98 10.82,17.37 11.43,17.37 12.04,17.98 12.04,18.29 11.58,18.75 11.58,20.27 12.8,21.49 v12.8,26.67 | v4.72,1.98 4.72,3.2 2.29,5.64 2.29,15.09 v5.03,17.83 | v21.64,30.18 21.64,35.97 19.05,38.56 19.05,48.16 21.03,50.14 27.28,50.14 27.89,50.75 27.89,51.05 23.93,55.02 23.16,55.02 19.51,58.67 14.02,58.67 12.8,57.45 IC1.3 12.65,57.3 10.82,57.3 8.69,55.17 7.62,55.17 | 7.62,55.17 v6.55,55.17 | 7.62,55.17 v7.62,45.41
+3V3_A  (via drill 0.3)
  Top 0.152: v26.21,45.57 26.21,44.5 IC7.4 | v27.89,42.22 27.43,42.22 27.28,42.06 22.71,42.06 22.4,42.37 C36.1 | 21.95,54.41 21.34,55.02 21.34,55.32 21.95,55.93 22.4,55.93 22.71,56.24 22.71,60.35 IC3.1 | 21.95,54.41 22.25,54.41 v23.93,56.08 27.43,59.59 C22.+ | IC5.8 8.69,8.84 8.69,8.08 8.38,7.77 8.38,6.71 C28.1 8.23,6.55 v8.23,5.18 | C30.+ 13.41,3.05 11.58,1.22 2.13,1.22 0.91,2.44 0.91,3.66 3.81,6.55 4.12,6.55 C27.1 4.27,6.55 v4.27,5.49 | v4.12,10.21 4.12,8.84 IC5.1 | C24.1 18.14,33.53 18.14,35.05 C23.1 17.98,35.05 17.98,36.27 17.22,37.03 IC4.24 17.22,37.19 18.29,38.25 | 18.29,38.25 18.59,38.56 IC4.25 | v11.28,40.23 10.21,40.23 IC4.9 | v8.99,35.66 7.16,33.83 C20.1 7.01,33.83 5.64,33.83 C19.1 5.49,33.68 4.12,32.31 4.12,28.5 JP3.1 | 18.29,38.25 13.87,42.67 v13.56,42.67 | v9.3,11.74 9.3,12.5 11.28,14.48 v11.28,18.14 | v21.95,54.1 21.95,54.41
  Bottom 0.152: v27.89,42.22 27.89,42.52 26.21,44.2 v26.21,45.57 26.21,48.16 28.5,50.44 28.5,51.51 v23.93,56.08 | 4.12,9.6 4.12,5.64 v4.27,5.49 4.57,5.18 v8.23,5.18 | 4.12,9.6 v4.12,10.21 | 4.12,9.6 5.79,9.6 7.92,11.74 v9.3,11.74 | v11.28,18.14 11.28,31.85 8.99,34.14 v8.99,35.66 9.75,36.42 9.75,38.71 v11.28,40.23 11.28,40.39 v13.56,42.67 13.56,44.65 21.95,53.03 v21.95,54.1
ADC_FM  (via drill 0.3)
  Top 0.152: IC7.1 28.19,44.5 28.19,46.33 28.5,46.63 C40.2 28.5,46.79 28.5,48.16 R19.1 28.5,48.31 27.74,49.07 27.74,50.29 v27.13,50.9 | v16,39.62 16.15,39.47 16.15,37.19 IC4.22
  Bottom 0.152: v16,39.62 16,46.02 21.64,51.66 26.36,51.66 v27.13,50.9
ADC_GATE
  Top 0.152: IC4.21 15.54,37.03 15.54,31.39 16,30.94 16,28.5 10.97,23.47 6.71,23.47 JP38.1
ADC_HARMONICS
  Top 0.152: 28.5,36.58 28.19,36.88 28.19,38.86 IC7.14 28.04,39.01 28.04,39.47 25.91,41.61 21.64,41.61 20.27,40.23 18.75,40.23 IC4.28 | 28.5,36.58 28.5,35.05 R20.1 | 28.5,36.58 C41.2
ADC_MODEL  (via drill 0.3)
  Top 0.152: v5.33,24.54 11.58,24.54 13.72,26.67 13.72,35.66 14.63,36.58 14.63,37.03 IC4.19
  Bottom 0.152: v5.33,24.54 3.2,24.54 2.13,23.47 1.52,23.47 JP35.1
ADC_MORPH
  Top 0.152: 23.32,36.58 24.08,37.34 24.08,38.86 IC7.8 24.08,39.01 23.47,39.62 18.75,39.62 IC4.27 | 23.32,36.58 23.32,35.05 R35.1 | 23.32,36.58 C49.2
ADC_TIMBRE  (via drill 0.3)
  Top 0.152: v15.24,38.25 15.24,37.19 IC4.20 | v17.68,26.82 17.68,25.91 17.37,25.6 17.37,21.64 v17.68,21.34 | v14.48,6.55 v14.48,13.26
  Bottom 0.152: v15.24,38.25 15.24,35.81 18.29,32.77 18.29,27.43 v17.68,26.82 | v17.68,21.34 17.68,16.46 v14.48,13.26 | v14.48,6.55 14.02,6.55 8.69,1.22 4.57,1.22 1.52,4.27 JP33.1
ADC_TRIG  (via drill 0.3)
  Top 0.152: v1.98,32.31 2.44,32.77 2.44,41.15 4.72,43.43 4.72,46.02 4.88,46.18 9.14,46.18 14.02,41.3 14.02,37.19 IC4.18
  Bottom 0.152: v1.98,32.31 5.33,28.96 5.33,25.45 6.25,24.54 7.16,24.54 7.77,23.93 7.77,22.86 7.01,22.1 5.33,22.1 JP39.1
ADC_V_OCT
  Top 0.152: IC7.7 24.08,44.5 24.08,45.87 23.32,46.63 C48.2 | IC4.26 18.59,39.17 17.98,39.17 16.76,40.39 16.76,43.28 19.51,46.02 22.55,46.02 23.16,46.63 C48.2 | R34.1 23.32,48.16 23.32,46.79 C48.2
AREF_-10  (via drill 0.3)
  Top 0.152: R23.2 28.5,49.83 28.5,50.44 27.28,51.66 25.45,51.66 23.62,49.83 23.32,49.83 R29.2 23.16,49.68 v21.03,47.55 | R27.2 R36.2 24.84,33.53 v24.84,30.48 | C50.1 20.73,14.02 19.36,14.02 R37.2 19.2,14.02 v18.14,14.02 | v22.25,12.8 22.71,13.26 22.71,13.72 IC9.2
  Bottom 0.152: 22.25,14.02 22.25,17.98 19.81,20.42 19.81,23.17 22.55,25.91 JP29.1 23.47,25.91 24.54,26.97 24.54,28.8 24.84,29.11 v24.84,30.48 24.84,38.71 20.88,42.67 20.88,44.2 21.03,44.35 v21.03,47.55 | 22.25,14.02 v22.25,12.8 | 22.25,14.02 v18.14,14.02
DAC_BCK  (via drill 0.3)
  Top 0.152: v17.53,40.54 17.68,40.69 18.59,40.69 IC4.29 | v19.81,32.16 19.81,26.06 v19.96,25.91 | v9.14,17.83 9.14,15.54 8.84,15.24 8.84,14.63 IC5.13
  Bottom 0.152: v17.53,40.54 17.53,34.44 v19.81,32.16 | v19.96,25.91 19.96,25.45 11.58,17.07 9.91,17.07 v9.14,17.83
DAC_DIN  (via drill 0.3)
  Top 0.152: v19.81,41.76 18.75,41.76 IC4.31 | v8.69,13.26 8.23,13.72 8.23,14.48 IC5.14
  Bottom 0.152: v19.81,41.76 19.81,38.25 22.4,35.66 22.4,29.26 20.88,27.74 20.88,25.45 v8.69,13.26
DAC_LRCK  (via drill 0.3)
  Top 0.152: v17.53,41.61 17.98,42.06 18.59,42.06 IC4.32 | v12.95,19.36 7.62,19.36 7.32,19.66 5.64,19.66 3.35,17.37 3.35,13.87 4.72,12.5 6.1,12.5 7.32,13.72 7.32,14.48 IC5.15
  Bottom 0.152: v17.53,41.61 18.75,40.39 18.75,34.14 20.57,32.31 20.57,27.43 19.2,26.06 19.2,25.15 13.41,19.36 v12.95,19.36
FREQ_ATT
  Top 0.152: IC4.15 12.65,37.19 12.65,37.64 12.34,37.95 11.43,37.95 10.82,37.34 10.82,32.61 6.71,28.5 JP19.1
FREQ_POT
  Top 0.152: JP15.1 2.74,27.13 2.74,35.36 4.27,36.88 5.64,36.88 8.38,39.62 10.06,39.62 IC4.10
GND  (via drill 0.3)
  Top 0.152: 14.63,33.53 14.63,32 | 14.63,33.53 14.63,35.05 C25.2 | 14.63,33.53 C9.2 | 16.46,35.05 16.61,35.2 16.61,37.03 IC4.23 | 16.46,35.05 16.46,33.53 | 16.46,35.05 C23.2 | 20.88,19.81 20.88,19.96 21.34,20.42 21.34,23.17 18.44,26.06 18.44,30.33 16.61,32.16 | 20.88,19.81 20.88,15.7 C50.2 | 16.61,32.16 16.46,32.31 16.46,33.53 | 16.46,33.53 C24.2 | 14.63,32 14.63,31.39 v15.24,30.79 | 16.61,32.16 v16.31,31.85 | 14.63,32 C26.2 | 19.51,4.42 19.51,3.05 C45.1 | 19.51,4.42 20.27,5.18 20.88,5.18 IC8.3 21.03,5.33 22.4,5.33 | 22.4,5.33 23.01,4.72 23.01,3.05 C35.2 | 23.62,8.99 23.62,8.69 23.16,8.23 C37.2 23.01,8.08 22.4,7.47 22.4,5.33 | 23.62,8.99 23.62,14.17 22.86,14.93 22.86,15.54 IC9.1 | 23.62,8.99 25.3,8.99 25.6,8.69 25.6,5.33 26.21,4.72 26.67,4.72 IC8.5 | C27.2 5.79,6.71 5.79,7.93 5.64,8.08 5.64,8.84 IC5.3 5.49,8.84 v5.49,10.67 | 5.79,6.1 5.79,6.55 C27.2 | 5.79,6.1 2.74,3.05 C7.- | C30.- 8.84,3.05 5.79,6.1 | 5.79,6.1 C27.2 | 10.06,6.86 IC5.10 IC5.9 9.3,8.84 9.3,10.82 8.53,11.58 8.53,12.19 | 10.06,6.86 10.06,6.71 C28.2 10.06,6.86 | 10.06,6.86 12.19,6.86 | C17.2 5.79,16.76 5.79,16.15 4.88,15.24 4.88,14.63 IC5.19 4.88,14.48 4.88,13.87 5.18,13.56 | 5.18,13.56 6.4,13.56 6.71,13.87 6.71,14.48 IC5.16 | C18.2 9.91,16.76 9.91,15.7 9.45,15.24 9.45,14.63 IC5.12 9.45,14.48 9.45,13.11 8.53,12.19 | 2.13,14.63 1.52,14.63 C31.2 2.13,14.63 | 3.96,12.8 4.57,12.19 8.53,12.19 | 3.96,12.8 2.13,14.63 | v4.88,13.26 5.18,13.56 | 3.96,12.8 v3.96,12.34 | 19.51,4.42 14.63,4.42 12.19,6.86 | 12.19,6.86 C33.2 | 20.88,19.81 13.56,19.81 12.5,20.88 v8.23,20.88 | 25.91,43.59 25.6,43.89 25.6,44.35 IC7.5 | 25.91,43.59 26.36,43.59 26.67,43.89 26.67,44.35 IC7.3
  Top 0.152: IC7.12 26.67,39.01 26.21,39.01 IC7.11 26.06,39.01 25.6,39.01 IC7.10 25.45,39.01 25.45,39.47 v24.23,40.69 22.4,40.69 C36.2 | v25.45,43.13 25.91,43.59 | 7.01,53.19 6.1,52.27 6.1,51.97 9.45,48.62 10.67,48.62 11.43,47.85 C10.2 11.58,47.7 12.04,47.24 12.04,45.72 IC4.47 12.19,45.57 12.19,45.11 12.5,44.81 13.26,44.81 13.56,45.11 13.56,45.57 IC4.44 13.72,45.72 13.72,46.79 14.48,47.55 14.78,47.55 15.54,46.79 v21.79,46.79 | 7.01,53.19 7.32,53.49 7.32,55.32 6.71,55.93 5.64,55.93 C15.2 | C14.1 3.5,46.63 3.5,45.11 3.66,44.96 Q1.2 3.66,44.81 1.37,42.52 1.37,40.54 Q1.4 1.37,40.39 1.68,40.08 1.68,38.71 C21.1 1.68,38.56 1.68,32.92 1.22,32.46 1.22,28.8 1.52,28.5 JP7.1 | C20.2 7.01,35.51 5.64,35.51 C19.2 5.49,35.51 5.03,35.51 v4.42,36.12 | v8.38,40.69 10.06,40.69 IC4.8 | 12.5,67.67 12.5,70.1 P1.3 | C22.- C4.- 27.43,68.88 29.11,70.56 29.11,77.27 28.5,77.88 24.84,77.88 24.08,77.11 24.08,76.2 21.95,74.07 20.42,74.07 17.53,71.17 P1.7 15.09,70.1 | 15.09,70.1 15.09,67.67 | 15.09,67.67 17.53,67.67 P1.8 | 15.09,67.67 P1.6 14.94,67.67 12.5,67.67 | 15.09,70.1 P1.5 | 12.5,67.67 P1.4 12.34,67.51 8.08,63.25 | 2.59,64.77 2.59,68.73 C5.+ | C13.2 22.71,62.94 22.71,61.87 21.34,60.5 IC3.2 21.34,59.59 19.05,57.3 19.05,56.84 18.29,56.08 16.46,56.08 15.39,57.15 | C2.2 8.38,62.94 9.45,61.87 9.45,60.5 C6.2 9.6,60.35 10.36,60.35 11.12,59.59 13.11,59.59 | 13.11,59.59 15.24,57.45 IC1.2 | 13.11,59.59 12.95,59.74 12.95,61.11 14.33,62.48 14.33,62.94 C1.2 | 15.39,57.15 15.24,57.3 IC1.2 | 2.59,64.77 6.55,64.77 8.08,63.25 | 8.08,63.25 8.23,63.09 C2.2 | 2.59,64.77 C3.- | 8.08,63.25 C2.2 | 7.01,53.19 8.99,51.21 9.45,51.21 15.39,57.15
  Top 0.152: 15.39,57.15 IC1.2 | 2.13,14.63 2.13,19.66 2.74,20.27 2.74,24.38 v2.44,24.69
  Bottom 0.152: v16.31,31.85 v15.24,30.79 | v5.49,10.67 3.96,12.19 v3.96,12.34 v4.88,13.26 5.79,14.17 5.79,18.44 7.01,19.66 7.16,19.66 7.77,20.27 7.77,20.42 v8.23,20.88 | v24.23,40.69 25.45,41.91 v25.45,43.13 v21.79,46.79 | JP6.1 7.16,43.89 | 7.16,43.89 8.38,42.67 v8.38,40.69 4.42,36.73 v4.42,36.12 1.22,32.92 1.22,32.16 1.52,31.85 JP7.1 1.52,28.35 2.74,27.13 2.74,25.45 2.44,25.15 v2.44,24.69 | 7.16,43.89 8.38,45.11 8.38,54.41 10.21,56.24 12.04,56.24 12.19,56.08 14.02,56.08 15.24,57.3 IC1.2
  other vias: 16.26,18.54 19.56,18.29 24.38,10.67 17.02,6.35 15.49,10.67 14.48,15.49 28.7,13.97 24.38,16 24.38,18.8 14.22,23.37 11.94,29.21 6.1,42.67 4.57,49.28 6.1,53.85 27.69,55.88 10.16,76.45 18.8,73.15 4.83,66.8 13.72,65.53 21.34,49.28 28.7,40.64 25.91,37.59 25.91,31.75 6.35,4.06
  pour Top: 0,0.04 30,0.04 30,79.04 0,79.04
  pour Bottom: 0,0.04 30,0.04 30,79.04 0,79.04
HARMONICS_POT  (via drill 0.3)
  Top 0.152: v9.75,34.29 10.06,34.59 10.06,38.56 IC4.12 | v20.57,23.01 v18.14,25.45 | v22.25,24.69 26.36,24.69 27.28,25.6 27.28,27.28 JP16.1
  Bottom 0.152: v9.75,34.29 9.75,33.83 v18.14,25.45 | v22.25,24.69 v20.57,23.01
JACKLIGHTS
  Top 0.152: JP59.1 20.27,76.66 20.27,76.2 16.31,72.24 13.72,72.24 11.89,74.07 8.08,74.07 5.49,76.66 4.62,76.66 JP2.2
  Bottom 0.152: 4.57,76.66 JP2.2
LEDS_SCK  (via drill 0.3)
  Top 0.152: v17.53,43.13 17.98,42.67 18.59,42.67 IC4.33 | v17.83,45.26 15.54,42.98 v15.24,42.98 | v25.3,55.93 v23.62,54.25
  Bottom 0.152: v17.53,43.13 17.53,44.96 v17.83,45.26 | v15.24,42.98 15.24,45.87 v23.62,54.25 | v25.3,55.93 25.3,76.66 JP11.1
LEDS_SIN  (via drill 0.3)
  Top 0.152: v19.96,44.04 19.66,43.74 18.75,43.74 IC4.35 | v19.96,52.58 v19.96,48.16 | v22.1,55.17 26.82,59.89 26.82,70.21 27.43,70.61 27.89,70.81 28.04,70.97 28.04,76.66 JP10.1
  Bottom 0.152: v19.96,48.16 v19.96,44.04 | v19.96,52.58 19.96,53.03 v22.1,55.17
LEDS_SS  (via drill 0.3)
  Top 0.152: v21.64,44.04 20.88,44.81 19.81,44.81 19.2,44.2 18.75,44.2 IC4.36
  Bottom 0.152: v21.64,44.04 21.64,42.37 24.08,39.93 24.38,39.93 26.21,41.76 26.21,43.28 24.23,45.26 24.23,46.63 28.19,50.6 28.19,51.21 24.08,55.32 23.77,55.32 23.16,55.93 23.16,71.63 24.54,73 24.54,74.98 22.86,76.66 JP12.1
MORPH_ATT  (via drill 0.3)
  Top 0.152: v9.45,28.19 12.04,30.79 12.04,37.03 IC4.14
  Bottom 0.152: v9.45,28.19 9.45,19.96 6.25,16.76 6.25,10.52 5.64,9.91 5.33,9.91 4.27,10.97 3.96,10.97 3.35,10.36 3.35,5.49 6.71,2.13 9.14,2.13 18.75,11.74 23.01,11.74 29.11,17.83 29.11,18.44 27.28,20.27 27.28,22.25 28.35,23.32 JP57.1
MORPH_POT  (via drill 0.3)
  Top 0.152: v11.28,39.17 10.21,39.17 IC4.11 | v17.22,32.46 17.22,32 19.2,30.02 19.2,25.76 22.86,22.1 26.36,22.1 27.28,23.01 27.28,24.84 28.35,25.91 JP18.1
  Bottom 0.152: v11.28,39.17 11.28,38.41 v17.22,32.46
N$1
  Top 0.152: 14.48,60.5 13.72,60.5 L1.2 | 14.48,60.5 17.07,63.09 C1.1 | 14.48,60.5 17.68,57.3 IC1.1
N$2
  Top 0.152: D1.+ 22.86,67.51 20.12,67.51 P1.10 20.12,67.67 20.12,70.1 P1.9
N$3
  Top 0.152: D2.- 7.16,67.51 9.91,67.51 P1.2 P1.1
N$6
  Top 0.152: IC5.2 4.72,8.84 4.72,8.08 4.42,7.77 2.44,7.77 1.52,8.69 C29.1
N$7
  Top 0.152: IC4.5 10.06,42.22 8.69,42.22 5.64,45.26 R5.1
N$8
  Top 0.152: IC4.6 10.06,41.61 7.16,41.61 5.64,40.08 R6.1
N$16
  Top 0.152: IC5.4 6.25,8.84 6.25,10.82 5.64,11.43 2.29,11.43 1.52,10.67 C29.2
N$29
  Top 0.152: Q1.3 1.37,44.96 1.68,45.26 1.68,46.63 C14.2 1.83,46.79 2.59,47.55 3.96,47.55 4.42,47.09 5.49,47.09 R5.2
N$30  (via drill 0.3)
  Top 0.152: R29.1 24.99,49.68 24.99,48.31 R34.2 24.99,48.16 24.99,46.79 C48.1 24.99,46.63 v24.99,45.57 24.99,44.5 IC7.6
  Bottom 0.152: v24.99,45.57 24.99,44.96 27.13,42.82 27.13,24.69 25.91,23.47 JP25.1
N$32
  Top 0.152: 24.99,36.58 24.99,38.86 IC7.9 | 23.32,33.53 24.84,35.05 R35.2 24.99,35.05 24.99,36.58 | 24.99,36.58 C49.1 | 23.32,33.53 23.32,31.09 25.91,28.5 JP23.1 | 23.32,33.53 R36.1
N$33
  Top 0.152: JP5.2 17.07,50.75 17.07,49.53 R10.1
N$34  (via drill 0.3)
  Top 0.152: IC7.2 27.43,44.5 27.43,46.18 26.98,46.63 C40.1 26.82,46.79 26.82,48.16 R19.2 26.82,48.31 26.82,49.68 R23.1 26.82,49.83 v25.76,50.9 | v12.34,20.12 7.32,20.12 JP21.1
  Bottom 0.152: v25.76,50.9 21.34,50.9 16.76,46.33 16.76,34.75 18.9,32.61 18.9,25.3 13.72,20.12 v12.34,20.12
N$35
  Top 0.152: R6.2 5.49,38.41 3.66,38.41 3.5,38.56 C21.2 3.5,38.71 3.66,38.86 3.66,40.39 Q1.1
N$38
  Top 0.152: F2.2 8.84,73.15 8.84,72.54 7.16,70.87 D2.+
N$40
  Top 0.152: 21.03,72.69 21.03,73.15 F1.2 21.03,72.69 | 21.03,72.69 22.86,70.87 D1.- | 18.14,64.16 18.29,64.01 18.29,62.03 17.98,61.72 17.22,61.72 16,60.5 F3.2 | 18.14,64.16 12.19,64.16 11.12,63.09 C2.1 11.12,62.94 11.73,62.33 11.73,60.5 L1.1 | 21.03,72.69 19.66,71.32 19.51,71.32 18.75,70.56 18.75,64.77 18.14,64.16
N$41
  Top 0.152: IC7.13 27.43,38.86 27.43,37.03 26.98,36.58 C41.1 26.82,36.58 26.82,35.05 R20.2 26.98,35.05 28.5,33.53 | 28.5,33.53 28.5,30.18 27.13,28.8 27.13,27.58 25.91,26.36 JP27.1 | 28.5,33.53 R27.1
N$42
  Top 0.152: F3.1 17.68,60.5 19.81,60.5 IC3.3 19.96,60.5 19.96,62.94 C13.1
N$43  (via drill 0.3)
  Top 0.152: v10.06,10.82 12.19,10.82 R11.2 | v8.38,10.36 7.47,9.45 7.47,8.84 IC5.6
  Bottom 0.152: v10.06,10.82 8.84,10.82 v8.38,10.36
N$46
  Top 0.152: C33.1 12.19,9.45 13.11,10.36 13.11,11.58 12.19,12.5 R11.1 R21.2
N$47
  Top 0.152: R12.1 24.69,1.52 24.69,3.05 C35.1 R16.2
N$48  (via drill 0.3)
  Top 0.152: v7.32,10.21 6.86,9.75 6.86,8.84 IC5.5 | v7.77,2.9 6.86,1.98 v5.94,1.98 | v3.05,12.8 1.52,12.8 C31.1
  Bottom 0.152: v7.32,10.21 7.32,7.01 8.99,5.33 8.99,4.11 v7.77,2.9 | v5.94,1.98 5.94,2.44 3.05,5.33 v3.05,12.8
N$51
  Top 0.152: R9.1 11.89,49.53 11.89,50.29 13.41,51.82 JP5.1
N$54
  Top 0.152: C18.1 7.32,16.76 6.1,15.54 5.79,15.54 5.64,15.39 5.64,14.63 IC5.18
N$55
  Top 0.152: R12.2 17.07,1.52 14.17,4.42 8.08,4.42 7.47,5.03 7.47,7.62 8.08,8.23 8.08,8.84 IC5.7
N$58
  Top 0.152: R28.2 28.35,9.6 28.35,8.23 C43.1 28.19,8.08 28.19,5.94 27.43,5.18 | 27.43,5.18 28.19,4.42 28.19,3.05 R16.1 | 27.43,5.18 26.82,5.18 IC8.6
N$60
  Top 0.152: IC8.7 26.67,5.94 26.21,5.94 25.91,6.25 25.91,7.47 26.52,8.08 C43.2 26.67,8.23 26.67,9.6 R28.1 26.52,9.75 26.52,16.46 25.91,17.07 JP53.1
N$62
  Top 0.152: R22.2 21.18,9.6 21.18,8.23 C42.1 21.18,8.08 21.18,7.47 21.79,6.86 21.79,6.25 21.49,5.94 21.03,5.94 IC8.2 20.88,5.94 19.96,5.94 16.61,9.3 16.61,12.04 12.19,16.46 R21.1
N$63
  Top 0.152: IC8.1 20.88,6.71 19.51,8.08 C42.2 19.51,8.23 19.51,9.6 R22.1 19.51,9.75 19.51,11.13 21.95,13.56 21.95,19.36 23.32,20.73 JP52.1
NORMALIZATION_PROBE  (via drill 0.3)
  Top 0.152: v20.88,41.76 20.12,41 19.66,41 19.51,41.15 18.75,41.15 IC4.30 | v20.88,38.1 20.88,25.15 22.55,23.47 23.32,23.47 JP31.1
  Bottom 0.152: v20.88,38.1 v20.88,41.76
RESET  (via drill 0.3)
  Top 0.152: v11.28,41.76 10.67,41.15 10.21,41.15 IC4.7 | v10.67,54.1 7.16,57.61 5.64,57.61 C15.1 5.49,57.76 4.12,57.76 R4.2 3.96,57.61 3.5,57.15 JP6.4
  Bottom 0.152: v11.28,41.76 11.28,51.82 10.67,52.43 v10.67,54.1
RX
  Top 0.152: IC4.46 12.65,45.72 12.65,48.77 13.41,49.53 R9.2
SW_1  (via drill 0.3)
  Top 0.152: v14.33,44.5 14.17,44.65 14.17,45.57 IC4.43 | v16.76,28.8 11.12,23.17 8.08,23.17 7.01,22.1 5.33,22.1 JP13.1
  Bottom 0.152: v14.33,44.5 14.33,36.27 17.98,32.61 17.98,30.02 v16.76,28.8
SW_2  (via drill 0.3)
  Top 0.152: v14.63,46.79 14.63,45.72 IC4.42 | v28.35,17.98 28.35,20.73 JP14.1
  Bottom 0.152: v14.63,46.79 14.63,48.92 11.43,52.12 11.43,55.17 10.67,55.93 10.36,55.93 9.6,55.17 9.6,52.43 9.91,52.12 9.91,40.23 8.23,38.56 8.23,33.53 10.97,30.79 10.97,21.03 6.55,16.61 6.55,14.48 8.53,12.5 21.64,12.5 22.1,12.04 22.4,12.04 v28.35,17.98
SWCLK
  Top 0.152: IC4.37 17.07,45.57 17.07,45.11 15.7,43.74 12.34,43.74 1.52,54.56 JP6.3
SWDIO  (via drill 0.3)
  Top 0.152: v6.86,52.12 8.08,50.9 9.6,50.9 12.04,53.34 26.36,53.34 29.41,50.29 29.41,44.65 27.13,42.37 25.3,42.37 24.38,43.28 18.75,43.28 IC4.34
  Bottom 0.152: v6.86,52.12 1.52,52.12 JP6.2
TIMBRE_ATT
  Top 0.152: JP56.1 5.79,25.91 4.57,24.69 3.5,24.69 2.9,25.3 2.9,26.52 3.5,27.13 4.42,27.13 5.33,28.04 5.33,28.96 10.52,34.14 10.52,37.49 11.28,38.25 12.65,38.25 13.11,37.8 13.11,37.19 IC4.16
TIMBRE_POT
  Top 0.152: IC4.13 11.58,37.03 11.58,31.7 7.01,27.13 5.33,27.13 4.12,25.91 JP17.1
TX
  Top 0.152: IC4.45 13.26,45.72 13.26,47.4 15.39,49.53 R10.2
VCC  (via drill 0.3)
  Top 0.152: 27.74,10.52 28.8,10.52 29.11,10.21 29.11,2.44 28.8,2.13 27.74,2.13 27.43,2.44 27.43,3.66 27.13,3.96 26.21,3.96 24.84,5.33 24.84,8.08 C37.1 | 27.74,10.52 27.43,10.21 27.43,7.32 26.82,6.71 IC8.8 | F1.1 v23.77,73.15 25.76,73.15 27.43,71.48 C4.+ | 27.74,10.52 27.74,16.15 v26.67,17.22 | v20.57,20.57 13.26,20.57 11.43,22.4 v10.21,22.4 | v9.14,51.97 9.14,54.71 v7.92,55.93
  Bottom 0.152: 7.92,72.24 22.86,72.24 v23.77,73.15 | 7.92,72.24 7.32,72.24 2.9,76.66 2.08,76.66 JP2.3 | v26.67,17.22 23.93,17.22 v20.57,20.57 | v10.21,22.4 10.21,31.09 7.92,33.38 7.92,39.32 9.14,40.54 v9.14,51.97 | 7.92,72.24 v7.92,55.93
VEE  (via drill 0.3)
  Top 0.152: F2.1 3.35,73.15 2.59,72.39 C5.- 2.44,72.39 2.44,70.71 1.83,70.1 1.83,59.89 3.2,58.52 7.16,58.52 v10.52,55.17 | v17.37,9.45 17.37,14.02 | 17.37,14.02 17.37,14.17 18.75,15.54 19.2,15.54 R37.1 | 21.18,4.57 21.03,4.57 IC8.4 21.18,4.57 | 21.18,4.57 v22.25,4.57 | 21.18,4.57 21.18,3.05 C45.2 | v7.16,36.58 v8.99,38.41 | v7.16,18.9 12.5,18.9 17.37,14.02
  Bottom 0.152: v22.25,4.57 v17.37,9.45 | v10.52,55.17 10.52,54.86 9.91,54.25 9.91,52.58 10.21,52.27 10.21,39.62 v8.99,38.41 | v7.16,36.58 7.16,29.57 8.99,27.74 8.99,20.73 v7.16,18.9

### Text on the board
bPlace: ON | OFF | JACK LIGHTS | ANTUMBRA | KNIT | V1.0 | WWW.ANTUMBRA.EU | REDESIGNED BY / DAVID SZEBENYI
bNames: cc-by-sa Olivier Gillet
tStop: Plaits | cc-by-sa | 2017. v5 | Olivier Gillet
